[IBIS Ver]   5.0
[File name]   rzg2ul_13mm.ibs
[File Rev]   1.02
[Date]   May 27, 2025
[Source]   From silicon level SPICE model at
|   Renesas Electronics Corporation.
[Notes]
|   RZG2UL_IBIS_MODEL
|(1) This IBIS file checked the format with ibischk7.
|   Format Error are 0 and Warning are 5.
|   The 5 Warnings can be ignored.
|(2) Temperature described Tj.
|   Tj[deg]
|   Typical   25.00
|   Minimum   125.00
|   Maximum   -40.00
|(3) History
|   Rev 1.02
|   New creation by Renesas Electronics
[Disclaimer]
   These IBIS models are provided "AS IS" with no warranty and RENESAS
   is not responsible for any problems this model may cause to the customers.
   These models are subject to change without any notice.
[Copyright]   Copyright (C) 2025, Renesas Electronics Corporation. ,
|   All Rights Reserved.
[Component]   R9A07G043Ux5GBG
[Manufacturer]  Renesas Electronics Corporation.
| IBIS	DATA
| date	:	2021.9.17
| product	:	RZ/G2UL(PKG-B)
| pin   :	361pin
| printed	by	Renesas	Electronics
[Package]
|   typ   min   max
R_pkg   0.22598   0.34368   0.13006
L_pkg   3.913e-9   6.179e-9   1.918e-9
C_pkg   5.506e-13   8.624e-13   3.59e-13
[Pin]   Signal_name   model_name   R_pin   L_pin   C_pin
A9   AUDIO_CLK1   gpio_33v   0.22861   4.147e-9   4.707e-13
B8   AUDIO_CLK2   gpio_33v   0.21663   3.755e-9   5.043e-13
AE22   BSCANP   inbuf_33v   0.23766   4.548e-9   5.913e-13
AD21   VSS   inbuf_33v   0.22763   3.912e-9   4.986e-13
AE11   CSI_CLKN   AS28FMIP0000_IN   0.20128   3.731e-9   5.503e-13
AD11   CSI_CLKP   AS28FMIP0000_IN   0.18569   3.345e-9   5.496e-13
AE12   CSI_DATA0_N   AS28FMIP0000_IN   0.20766   3.838e-9   5.441e-13
AD12   CSI_DATA0_P   AS28FMIP0000_IN   0.19122   3.829e-9   5.488e-13
AE10   CSI_DATA1_N   AS28FMIP0000_IN   0.21307   4.036e-9   5.315e-13
AD10   CSI_DATA1_P   AS28FMIP0000_IN   0.19753   3.631e-9   5.495e-13
AE13   CSI_DATA2_N   AS28FMIP0000_IN   0.19175   3.578e-9   5.136e-13
AD13   CSI_DATA2_P   AS28FMIP0000_IN   0.18647   3.071e-9   4.943e-13
AE9   CSI_DATA3_N   AS28FMIP0000_IN   0.21591   3.771e-9   4.931e-13
AD9   CSI_DATA3_P   AS28FMIP0000_IN   0.19652   3.518e-9   5.449e-13
E25   DDR_ADDR0   DDR_ADRCNT   0.30852   5.269e-9   6.159e-13
K25   DDR_ADDR1   DDR_ADRCNT   0.29634   4.554e-9   5.505e-13
C25   DDR_ADDR2   DDR_ADRCNT   0.26285   5.286e-9   6.163e-13
C24   DDR_ADDR3   DDR_ADRCNT   0.28989   5.352e-9   6.454e-13
K23   DDR_ADDR4   DDR_ADRCNT   0.17693   2.994e-9   6.191e-13
B25   DDR_ADDR5   DDR_ADRCNT   0.33272   6.113e-9   6.962e-13
J25   DDR_ADDR6   DDR_ADRCNT   0.27229   4.79e-9   4.998e-13
A24   DDR_ADDR7   DDR_ADRCNT   0.34368   5.378e-9   7.14e-13
F25   DDR_ADDR8   DDR_ADRCNT   0.29546   5.204e-9   6.227e-13
B24   DDR_ADDR9   DDR_ADRCNT   0.26012   4.939e-9   7.012e-13
P23   DDR_ADDR10   DDR_ADRCNT   0.18289   2.726e-9   6.091e-13
H25   DDR_ADDR11   DDR_ADRCNT   0.22105   3.873e-9   4.949e-13
N23   DDR_ADDR12   DDR_ADRCNT   0.17797   2.693e-9   7.079e-13
D23   DDR_ADDR13   DDR_ADRCNT   0.22666   3.81e-9   5.753e-13
H23   DDR_ADDR14   DDR_ADRCNT   0.18025   2.93e-9   8.022e-13
D25   DDR_ADDR15   DDR_ADRCNT   0.29085   4.879e-9   6.257e-13
E24   DDR_BA0   DDR_ADRCNT   0.22101   3.606e-9   8.624e-13
L24   DDR_BA1   DDR_ADRCNT   0.2406   4.046e-9   5.626e-13
F23   DDR_BA2   DDR_ADRCNT   0.19749   3.016e-9   5.408e-13
A23   DDR_CALIBRATION   DDR_ADRCNT   0.27572   5.06e-9   6.049e-13
J24   DDR_CAS#   DDR_ADRCNT   0.19882   3.454e-9   5.111e-13
M25   DDR_CKE   DDR_ADRCNT   0.28365   4.337e-9   5.383e-13
P24   DDR_CLK_N   DDR_ADRCNT   0.2062   3.263e-9   4.953e-13
P25   DDR_CLK_P   DDR_ADRCNT   0.22344   3.65e-9   5.223e-13
N24   DDR_CS0#   DDR_ADRCNT   0.26763   3.955e-9   4.808e-13
L23   DDR_CS1#   DDR_ADRCNT   0.17047   2.819e-9   5.72e-13
U23   DDR_DM0   DDR_DQDMDQS   0.18554   2.794e-9   6.509e-13
Y24   DDR_DM1   DDR_DQDMDQS   0.28328   4.288e-9   6.595e-13
T25   DDR_DQ0   DDR_DQDMDQS   0.2478   4.283e-9   5.606e-13
W24   DDR_DQ1   DDR_DQDMDQS   0.23177   3.721e-9   4.888e-13
R24   DDR_DQ2   DDR_DQDMDQS   0.21916   3.48e-9   4.656e-13
Y25   DDR_DQ3   DDR_DQDMDQS   0.32654   4.752e-9   5.881e-13
T24   DDR_DQ4   DDR_DQDMDQS   0.27525   3.952e-9   5.711e-13
U25   DDR_DQ5   DDR_DQDMDQS   0.26125   4.103e-9   4.181e-13
R25   DDR_DQ6   DDR_DQDMDQS   0.28132   4.458e-9   4.363e-13
T23   DDR_DQ7   DDR_DQDMDQS   0.18032   2.637e-9   4.866e-13
AD24   DDR_DQ8   DDR_DQDMDQS   0.32838   4.655e-9   6.905e-13
AA24   DDR_DQ9   DDR_DQDMDQS   0.2742   4.67e-9   5.683e-13
W23   DDR_DQ10   DDR_DQDMDQS   0.18485   2.966e-9   4.618e-13
AD25   DDR_DQ11   DDR_DQDMDQS   0.27727   4.493e-9   7.8e-13
AD23   DDR_DQ12   DDR_DQDMDQS   0.25366   4.031e-9   7.58e-13
AA23   DDR_DQ13   DDR_DQDMDQS   0.20546   3.203e-9   7.392e-13
AC24   DDR_DQ14   DDR_DQDMDQS   0.30091   4.578e-9   7.764e-13
AE24   DDR_DQ15   DDR_DQDMDQS   0.33205   4.835e-9   5.793e-13
V24   DDR_DQS0_N   DDR_DQDMDQS   0.2145   3.127e-9   7.214e-13
V25   DDR_DQS0_P   DDR_DQDMDQS   0.23258   3.363e-9   6.777e-13
AB25   DDR_DQS1_N   DDR_DQDMDQS   0.26811   4.843e-9   6.631e-13
AB24   DDR_DQS1_P   DDR_DQDMDQS   0.27051   4.409e-9   7.234e-13
M24   DDR_ODT0   DDR_ADRCNT   0.22209   3.696e-9   5.376e-13
L25   DDR_ODT1   DDR_ADRCNT   0.27722   4.972e-9   5.408e-13
H24   DDR_RAS#   DDR_ADRCNT   0.26066   4.61e-9   5.523e-13
B23   DDR_RESET#   DDR_ADRCNT   0.31098   5.139e-9   6.32e-13
G25   DDR_WE#   DDR_ADRCNT   0.24637   4.632e-9   5.755e-13
Y19   DEBUGEN   inbuf_33v   0.15054   2.54e-9   6.669e-13
A10   DISP_CLK   gpio_33v   0.19853   3.939e-9   4.928e-13
B10   DISP_DATA0   gpio_33v   0.20629   3.552e-9   4.659e-13
A11   DISP_DATA1   gpio_33v   0.23075   3.819e-9   4.912e-13
B11   DISP_DATA2   gpio_33v   0.21122   3.381e-9   4.594e-13
A12   DISP_DATA3   gpio_33v   0.23395   3.581e-9   4.354e-13
B12   DISP_DATA4   gpio_33v   0.17421   3.057e-9   4.43e-13
C11   DISP_DATA5   gpio_33v   0.15695   2.26e-9   4.267e-13
C12   DISP_DATA6   gpio_33v   0.19989   3.05e-9   5.531e-13
C13   DISP_DATA7   gpio_33v   0.19809   3.019e-9   4.691e-13
A13   DISP_DATA8   gpio_33v   0.22642   3.908e-9   4.72e-13
B13   DISP_DATA9   gpio_33v   0.18059   3.095e-9   4.947e-13
A14   DISP_DATA10   gpio_33v   0.22656   3.822e-9   4.855e-13
C14   DISP_DATA11   gpio_33v   0.14189   2.292e-9   5.438e-13
B14   DISP_DATA12   gpio_33v   0.20803   3.339e-9   4.987e-13
C15   DISP_DATA13   gpio_33v   0.19625   3.149e-9   5.702e-13
A15   DISP_DATA14   gpio_33v   0.22045   3.914e-9   5.069e-13
F16   DISP_DATA15   gpio_33v   0.13006   1.918e-9   4.682e-13
B15   DISP_DATA16   gpio_33v   0.17178   3.267e-9   4.714e-13
C16   DISP_DATA17   gpio_33v   0.13851   2.371e-9   4.245e-13
A16   DISP_DATA18   gpio_33v   0.22064   3.986e-9   5.073e-13
B16   DISP_DATA19   gpio_33v   0.19052   3.137e-9   4.751e-13
A17   DISP_DATA20   gpio_33v   0.22782   4.166e-9   5.222e-13
B17   DISP_DATA21   gpio_33v   0.20624   3.572e-9   4.594e-13
C17   DISP_DATA22   gpio_33v   0.20862   3.611e-9   5.4e-13
C20   DISP_DATA23   gpio_33v   0.21051   3.694e-9   4.442e-13
C9   DISP_DE   gpio_33v   0.15116   2.627e-9   4.184e-13
B9   DISP_HSYNC   gpio_33v   0.2102   3.714e-9   4.29e-13
C10   DISP_VSYNC   gpio_33v   0.20786   3.501e-9   4.613e-13
P1   ET0_LINKSTA   rgmii_RIP_BI_SDS_1833V_NC   0.23928   4.222e-9   5.233e-13
T3   ET0_MDC   rgmii_RIP_BI_SDS_1833V_NC   0.21992   3.494e-9   5.227e-13
T2   ET0_MDIO   rgmii_RIP_BI_SDS_1833V_NC   0.21286   3.468e-9   5.939e-13
N3   ET0_RXC/RX_CLK   rgmii_RIP_BI_SDS_1833V_NC   0.21486   3.382e-9   5.835e-13
P2   ET0_RXD0   rgmii_RIP_BI_SDS_1833V_NC   0.1839   3.418e-9   4.518e-13
R3   ET0_RXD1   rgmii_RIP_BI_SDS_1833V_NC   0.21332   3.578e-9   5.481e-13
R2   ET0_RXD2   rgmii_RIP_BI_SDS_1833V_NC   0.22457   3.76e-9   5.597e-13
R1   ET0_RXD3   rgmii_RIP_BI_SDS_1833V_NC   0.23988   4.317e-9   5.185e-13
N1   ET0_RX_CTL/RX_DV   rgmii_RIP_BI_SDS_1833V_NC   0.23729   4.049e-9   5.049e-13
N2   ET0_RX_ERR   rgmii_RIP_BI_SDS_1833V_NC   0.21881   3.664e-9   4.935e-13
M2   ET0_TXC/TX_CLK   rgmii_RIP_BI_SDS_1833V_NC   0.20357   3.313e-9   4.826e-13
L1   ET0_TXD0   rgmii_RIP_BI_SDS_1833V_NC   0.24019   4.155e-9   5.204e-13
L2   ET0_TXD1   rgmii_RIP_BI_SDS_1833V_NC   0.22097   3.526e-9   5.78e-13
K1   ET0_TXD2   rgmii_RIP_BI_SDS_1833V_NC   0.23897   4.163e-9   5.179e-13
K2   ET0_TXD3   rgmii_RIP_BI_SDS_1833V_NC   0.22361   3.659e-9   5.463e-13
M3   ET0_TX_COL   rgmii_RIP_BI_SDS_1833V_NC   0.13984   2.506e-9   4.252e-13
M6   ET0_TX_CRS   rgmii_RIP_BI_SDS_1833V_NC   0.13124   2.049e-9   4.926e-13
M1   ET0_TX_CTL/TX_EN   rgmii_RIP_BI_SDS_1833V_NC   0.23547   4.139e-9   5.272e-13
K6   ET0_TX_ERR   rgmii_RIP_BI_SDS_1833V_NC   0.2133   3.521e-9   5.968e-13
AC19   ET1_LINKSTA   rgmii_RIP_BI_SDS_1833V_NC   0.21229   3.367e-9   5.938e-13
AC20   ET1_MDC   rgmii_RIP_BI_SDS_1833V_NC   0.19485   3.192e-9   4.294e-13
AE21   ET1_MDIO   rgmii_RIP_BI_SDS_1833V_NC   0.24993   4.505e-9   5.2e-13
AC17   ET1_RXC/RX_CLK   rgmii_RIP_BI_SDS_1833V_NC   0.19068   3.173e-9   5.904e-13
AE19   ET1_RXD0   rgmii_RIP_BI_SDS_1833V_NC   0.2318   4.258e-9   5.507e-13
AD19   ET1_RXD1   rgmii_RIP_BI_SDS_1833V_NC   0.21543   3.788e-9   5.39e-13
AE20   ET1_RXD2   rgmii_RIP_BI_SDS_1833V_NC   0.23799   4.307e-9   5.456e-13
AD20   ET1_RXD3   rgmii_RIP_BI_SDS_1833V_NC   0.22453   3.747e-9   5.686e-13
AC18   ET1_RX_CTL/RX_DV   rgmii_RIP_BI_SDS_1833V_NC   0.14167   2.338e-9   4.536e-13
AD18   ET1_RX_ERR   rgmii_RIP_BI_SDS_1833V_NC   0.2107   3.683e-9   5.402e-13
AE18   ET1_TXC/TX_CLK   rgmii_RIP_BI_SDS_1833V_NC   0.22618   4.132e-9   4.835e-13
AD16   ET1_TXD0   rgmii_RIP_BI_SDS_1833V_NC   0.1911   3.153e-9   4.595e-13
AE16   ET1_TXD1   rgmii_RIP_BI_SDS_1833V_NC   0.22095   4.002e-9   4.821e-13
AD15   ET1_TXD2   rgmii_RIP_BI_SDS_1833V_NC   0.20437   3.453e-9   4.809e-13
AE15   ET1_TXD3   rgmii_RIP_BI_SDS_1833V_NC   0.20919   3.458e-9   4.123e-13
AC16   ET1_TX_COL   rgmii_RIP_BI_SDS_1833V_NC   0.1327   2.314e-9   4.305e-13
AC15   ET1_TX_CRS   rgmii_RIP_BI_SDS_1833V_NC   0.14353   2.264e-9   4.933e-13
AD17   ET1_TX_CTL/TX_EN   rgmii_RIP_BI_SDS_1833V_NC   0.20566   3.594e-9   4.827e-13
AE17   ET1_TX_ERR   rgmii_RIP_BI_SDS_1833V_NC   0.22147   4.045e-9   4.995e-13
Y3   EXCLK   inbuf_33v   0.18247   2.935e-9   4.861e-13
B22   IRQ6   gpio_33v   0.238   4.391e-9   4.568e-13
A21   IRQ7   gpio_33v   0.22295   4.52e-9   5.478e-13
G6   MD_BOOT0   inbuf_33v   0.17061   2.786e-9   5.253e-13
C5   MD_BOOT1   inbuf_33v   0.20696   3.408e-9   4.625e-13
C4   MD_BOOT2   inbuf_33v   0.21541   3.666e-9   4.748e-13
F20   MD_CLKS   inbuf_33v   0.20617   3.517e-9   5.444e-13
A22   MD_OSCDRV0   inbuf_33v   0.25713   4.841e-9   5.306e-13
C21   MD_OSCDRV1   inbuf_33v   0.17909   3.207e-9   3.792e-13
AA2   NMI   gpio_33v   0.23155   4.205e-9   7.23e-13
B2   NC   sdio_STP_BI_016_1833V_SD3   0.26124   4.797e-9   5.818e-13
A4   NC   sdio_STP_BI_016_1833V_SD3   0.26691   5.034e-9   5.827e-13
B4   NC   sdio_STP_BI_016_1833V_SD3   0.25349   4.576e-9   6.25e-13
A3   NC   sdio_STP_BI_016_1833V_SD3   0.25227   4.987e-9   5.937e-13
B3   NC   sdio_STP_BI_016_1833V_SD3   0.26984   4.809e-9   6.384e-13
A2   NC   sdio_STP_BI_016_1833V_SD3   0.29359   5.578e-9   6.773e-13
AC3   P5_1   gpio_33v   0.16462   3.407e-9   4.695e-13
AB2   P6_2   gpio_33v   0.27733   6.179e-9   5.998e-13
AC1   P6_3   gpio_33v   0.25661   5.108e-9   5.885e-13
AC2   P6_4   gpio_33v   0.23412   3.923e-9   6.024e-13
W2   PRST#   gpio_33v   0.13355   3.131e-9   5.388e-13
C7   QSPI0_IO0   sdio_STP_BI_016_1833V_SD3   0.21696   3.457e-9   5.407e-13
A5   QSPI0_IO1   sdio_STP_BI_016_1833V_SD3   0.25155   4.652e-9   5.678e-13
B7   QSPI0_IO2   sdio_STP_BI_016_1833V_SD3   0.22587   3.789e-9   5.737e-13
C6   QSPI0_IO3   sdio_STP_BI_016_1833V_SD3   0.22339   3.646e-9   5.416e-13
B6   QSPI0_SPCLK   sdio_STP_BI_016_1833V_SD3   0.20303   3.787e-9   5.345e-13
B5   QSPI0_SSL   sdio_STP_BI_016_1833V_SD3   0.24229   4.387e-9   5.664e-13
A7   QSPI_RESET#   sdio_STP_BI_016_1833V_SD3   0.24456   4.339e-9   5.523e-13
A6   QSPI_WP#   sdio_STP_BI_016_1833V_SD3   0.25587   4.507e-9   5.749e-13
B19   RIIC0_SCL   iic_33v   0.20428   3.35e-9   4.125e-13
B20   RIIC0_SDA   iic_33v   0.23614   3.967e-9   5.251e-13
A19   RIIC1_SCL   iic_33v   0.24373   4.293e-9   4.502e-13
A20   RIIC1_SDA   iic_33v   0.25488   4.429e-9   5.437e-13
B1   SD0_CD   gpio_33v   0.27618   5.469e-9   6.12e-13
G1   SD0_CLK   sdio_STP_BI_016_1833V_SD3   0.26669   4.94e-9   5.992e-13
E2   SD0_CMD   sdio_STP_BI_016_1833V_SD3   0.24036   4.423e-9   5.822e-13
F1   SD0_DATA0   sdio_STP_BI_016_1833V_SD3   0.28096   5.207e-9   5.788e-13
H3   SD0_DATA1   sdio_STP_BI_016_1833V_SD3   0.21572   3.747e-9   7.649e-13
F2   SD0_DATA2   sdio_STP_BI_016_1833V_SD3   0.23704   4.353e-9   6.061e-13
D2   SD0_DATA3   sdio_STP_BI_016_1833V_SD3   0.22699   4.002e-9   6.391e-13
E1   SD0_DATA4   sdio_STP_BI_016_1833V_SD3   0.252   4.728e-9   6.238e-13
D1   SD0_DATA5   sdio_STP_BI_016_1833V_SD3   0.25925   4.933e-9   5.889e-13
E3   SD0_DATA6   sdio_STP_BI_016_1833V_SD3   0.22365   3.793e-9   7.306e-13
F3   SD0_DATA7   sdio_STP_BI_016_1833V_SD3   0.2175   3.618e-9   5.977e-13
C1   SD0_RST#   sdio_STP_BI_016_1833V_SD3   0.2641   5.004e-9   6.63e-13
C2   SD0_WP   gpio_33v   0.25951   4.981e-9   5.668e-13
D3   SD1_CD   gpio_33v   0.21151   3.733e-9   5.544e-13
G2   SD1_CLK   sdio_STP_BI_016_1833V_SD3   0.2266   3.877e-9   5.907e-13
H6   SD1_CMD   sdio_STP_BI_016_1833V_SD3   0.21716   3.71e-9   7.013e-13
H2   SD1_DATA0   sdio_STP_BI_016_1833V_SD3   0.23134   3.903e-9   5.261e-13
J3   SD1_DATA1   sdio_STP_BI_016_1833V_SD3   0.15703   2.653e-9   5.032e-13
J1   SD1_DATA2   sdio_STP_BI_016_1833V_SD3   0.23838   4.194e-9   5.026e-13
J2   SD1_DATA3   sdio_STP_BI_016_1833V_SD3   0.22062   3.657e-9   5.246e-13
C3   SD1_WP   gpio_33v   0.18174   3.832e-9   5.818e-13
U2   TCK/SWDCLK   inbuf_18v   0.23262   3.792e-9   3.996e-13
W1   TDI   inbuf_18v   0.26173   4.632e-9   5.884e-13
V2   TDO   gpio_18v   0.23571   3.957e-9   5.511e-13
AD22   VSS   inbuf_33v   0.24153   4.382e-9   4.981e-13
U1   TMS/SWDIO   gpio_18v   0.24779   4.278e-9   5.03e-13
V1   TRST#   inbuf_18v   0.22355   4.318e-9   5.309e-13
AE6   USB0_DM   as28fus20002vwbp1hs_dm   0.23395   3.919e-9   5.907e-13
AD6   USB0_DP   as28fus20002vwbp1hs_dp   0.21645   3.683e-9   6.102e-13
AB3   USB0_OTG_EXICEN   gpio_33v   0.21864   3.991e-9   6.97e-13
AD2   USB0_OTG_ID   gpio_33v   0.25189   4.972e-9   6.132e-13
AE3   USB0_OVRCUR   gpio_33v   0.26986   5.24e-9   6.012e-13
AD3   USB0_VBUSEN   gpio_33v   0.24994   4.648e-9   5.443e-13
AD8   USB0_VBUSIN   iic_33v   0.2033   3.727e-9   3.59e-13
AE5   USB1_DM   as28fus20002vwbp1hs_dm   0.24031   3.992e-9   5.792e-13
AD5   USB1_DP   as28fus20002vwbp1hs_dp   0.23092   3.546e-9   6.05e-13
AE2   USB1_OVRCUR   gpio_33v   0.23373   5.484e-9   6.009e-13
AD1   USB1_VBUSEN   gpio_33v   0.29109   5.779e-9   7.063e-13
B21   WDTOVF_PERROUT#   gpio_33v   0.20442   3.983e-9   5.655e-13
[Series Pin Mapping]   pin_2   model_name
AD11 AE11 AS28FMIP0000_TERM
AD12 AE12 AS28FMIP0000_TERM
AD10 AE10 AS28FMIP0000_TERM
AD13 AE13 AS28FMIP0000_TERM
AD9 AE9 AS28FMIP0000_TERM
[Diff Pin] inv_pin   vdiff   tdelay_typ   tdelay_min   tdelay_max
| The '+' pin is Diff_pin and the '-' pin is the inv_pin
| Receiver Vth = +/-100mV
|PAD_P   PAD_N   0.07   0   0   0
AD11 AE11 0.07 0 0 0
AD12 AE12 0.07 0 0 0
AD10 AE10 0.07 0 0 0
AD13 AE13 0.07 0 0 0
AD9 AE9 0.07 0 0 0
|[Diff pin]  inv_pin  vdiff   tdelay_typ   tdelay_min   tdelay_max
|DP   DM   100.000mV  0.0s   0.0s   0.0s
AD6 AE6 100mV 0 0 0
AD5 AE5 100mV 0 0 0
[Model Selector] gpio_33v
gpio_33v_12m_fast  SRP_BI_SDS_33V_STB_33V_e2e1_11_SR1
gpio_33v_12m_slow  SRP_BI_SDS_33V_STB_33V_e2e1_11_SR0
gpio_33v_2m_fast   SRP_BI_SDS_33V_STB_33V_e2e1_00_SR1
gpio_33v_2m_slow   SRP_BI_SDS_33V_STB_33V_e2e1_00_SR0
gpio_33v_4m_fast   SRP_BI_SDS_33V_STB_33V_e2e1_01_SR1
gpio_33v_4m_slow   SRP_BI_SDS_33V_STB_33V_e2e1_01_SR0
gpio_33v_8m_fast   SRP_BI_SDS_33V_STB_33V_e2e1_10_SR1
gpio_33v_8m_slow   SRP_BI_SDS_33V_STB_33V_e2e1_10_SR0
[Model Selector] gpio_18v
gpio_18v_12m_fast  SRP_BI_SDS_33V_STB_18V_e2e1_11_SR1
gpio_18v_12m_slow  SRP_BI_SDS_33V_STB_18V_e2e1_11_SR0
gpio_18v_2m_fast   SRP_BI_SDS_33V_STB_18V_e2e1_00_SR1
gpio_18v_2m_slow   SRP_BI_SDS_33V_STB_18V_e2e1_00_SR0
gpio_18v_4m_fast   SRP_BI_SDS_33V_STB_18V_e2e1_01_SR1
gpio_18v_4m_slow   SRP_BI_SDS_33V_STB_18V_e2e1_01_SR0
gpio_18v_8m_fast   SRP_BI_SDS_33V_STB_18V_e2e1_10_SR1
gpio_18v_8m_slow   SRP_BI_SDS_33V_STB_18V_e2e1_10_SR0
[Model Selector] sdio_STP_BI_016_1833V_SD3
sdio_18v_33_fast   STP_BI_016_1833V_SD3_18V_e2e1_00_SR0
sdio_18v_33_slow   STP_BI_016_1833V_SD3_18V_e2e1_00_SR0
sdio_18v_50_fast   STP_BI_016_1833V_SD3_18V_e2e1_01_SR0
sdio_18v_50_slow   STP_BI_016_1833V_SD3_18V_e2e1_01_SR0
sdio_18v_66_fast   STP_BI_016_1833V_SD3_18V_e2e1_10_SR0
sdio_18v_66_slow   STP_BI_016_1833V_SD3_18V_e2e1_10_SR0
sdio_18v_100_fast  STP_BI_016_1833V_SD3_18V_e2e1_11_SR0
sdio_18v_100_slow  STP_BI_016_1833V_SD3_18V_e2e1_11_SR0
sdio_33v_5_fast   STP_BI_016_1833V_SD3_33V_e2e1_11_SR0
sdio_33v_5_slow   STP_BI_016_1833V_SD3_33V_e2e1_11_SR0
sdio_33v_12_fast  STP_BI_016_1833V_SD3_33V_e2e1_10_SR0
sdio_33v_12_slow  STP_BI_016_1833V_SD3_33V_e2e1_10_SR0
sdio_33v_26_fast  STP_BI_016_1833V_SD3_33V_e2e1_01_SR0
sdio_33v_26_slow  STP_BI_016_1833V_SD3_33V_e2e1_01_SR0
sdio_33v_40_fast  STP_BI_016_1833V_SD3_33V_e2e1_00_SR0
sdio_33v_40_slow  STP_BI_016_1833V_SD3_33V_e2e1_00_SR0
[Model Selector] rgmii_RIP_BI_SDS_1833V_NC
rgmii_18v   RIP_BI_SDS_1833V_NC_18
rgmii_25v   RIP_BI_SDS_1833V_NC_25
rgmii_33v   RIP_BI_SDS_1833V_NC_33
[Model Selector] DDR_ADRCNT
PAD_60_0_USEIO_ddr4_0p5   Z0=60-Ohm Driver   ODT disable
PAD_60_0_USEIO_ddr3l   Z0=60-Ohm Driver   ODT disable
PAD_60_0_USEIO_ddr3   Z0=60-Ohm Driver   ODT disable
[Model Selector] DDR_DQDMDQS
PAD_40_120_USEIO_ddr4_0p8   Z0=40-Ohm Driver   120-Ohm Pull-up
PAD_40_80_USEIO_ddr4_0p8   Z0=40-Ohm Driver   80-Ohm Pull-up
PAD_40_60_USEIO_ddr4_0p8   Z0=40-Ohm Driver   60-Ohm Pull-up
PAD_40_48_USEIO_ddr4_0p8   Z0=40-Ohm Driver   48-Ohm Pull-up
PAD_40_40_USEIO_ddr4_0p8   Z0=40-Ohm Driver   40-Ohm Pull-up
PAD_34_0_USEIO_ddr4_0p8   Z0=34-Ohm Driver   ODT disable
PAD_48_0_USEIO_ddr4_0p8   Z0=48-Ohm Driver   ODT disable
PAD_60_0_USEIO_ddr4_0p8   Z0=60-Ohm Driver   ODT disable
PAD_40_120_USEIO_ddr3l   Z0=40-Ohm Driver   120-Ohm equivalent termination
PAD_40_60_USEIO_ddr3l   Z0=40-Ohm Driver   60-Ohm equivalent termination
PAD_40_40_USEIO_ddr3l   Z0=40-Ohm Driver   40-Ohm equivalent termination
PAD_34_0_USEIO_ddr3l   Z0=34-Ohm Driver   ODT disable
PAD_48_0_USEIO_ddr3l   Z0=48-Ohm Driver   ODT disable
PAD_60_0_USEIO_ddr3l   Z0=60-Ohm Driver   ODT disable
PAD_40_120_USEIO_ddr3   Z0=40-Ohm Driver   120-Ohm equivalent termination
PAD_40_60_USEIO_ddr3   Z0=40-Ohm Driver   60-Ohm equivalent termination
PAD_40_40_USEIO_ddr3   Z0=40-Ohm Driver   40-Ohm equivalent termination
PAD_34_0_USEIO_ddr3   Z0=34-Ohm Driver   ODT disable
PAD_48_0_USEIO_ddr3   Z0=48-Ohm Driver   ODT disable
PAD_60_0_USEIO_ddr3   Z0=60-Ohm Driver   ODT disable
|   Model AS28FMIP0000_TERM
[Model]   AS28FMIP0000_TERM
Model_type   Series
Polarity   Non-Inverting
C_comp   0.0pF   0.0pF   0.0pF
[Temperature Range] 25   125   -40
[Voltage Range]   1.8   1.65   1.95
| Resistance   ohm(typ)   ohm(min)   ohm(max)
[R Series]   100   80   125
| Models and submodels in the file (342): gpio_33v_12m_fast (I/O), gpio_33v_12m_slow (I/O), gpio_33v_2m_fast (I/O), gpio_33v_2m_slow (I/O), gpio_33v_4m_fast (I/O), gpio_33v_4m_slow (I/O), gpio_33v_8m_fast (I/O), gpio_33v_8m_slow (I/O), gpio_18v_12m_fast (I/O), gpio_18v_12m_slow (I/O), gpio_18v_2m_fast (I/O), gpio_18v_2m_slow (I/O), gpio_18v_4m_fast (I/O), gpio_18v_4m_slow (I/O), gpio_18v_8m_fast (I/O), gpio_18v_8m_slow (I/O), sdio_18v_33_fast (I/O), sdio_18v_33_slow (I/O), sdio_18v_50_fast (I/O), sdio_18v_50_slow (I/O), sdio_18v_66_fast (I/O), sdio_18v_66_slow (I/O), sdio_18v_100_fast (I/O), sdio_18v_100_slow (I/O), sdio_33v_5_fast (I/O), sdio_33v_5_slow (I/O), sdio_33v_12_fast (I/O), sdio_33v_12_slow (I/O), sdio_33v_26_fast (I/O), sdio_33v_26_slow (I/O), sdio_33v_40_fast (I/O), sdio_33v_40_slow (I/O), rgmii_18v (I/O), rgmii_25v (I/O), rgmii_33v (I/O), iic_33v (I/O_open_drain), inbuf_18v (Input), inbuf_33v (Input), AS28FMIP0000_IN (Input), as28fus20002vwbp1hs_dp (I/O), as28fus20002vwbp1hs_dm (I/O), AS28FMIP0000_TERM (Series), PAD_60_0_USEIO_ddr3 (I/O), PAD_60_120_USEIO_ddr3 (I/O), PAD_60_120_ddr3_T (Dynamic_clamp), PAD_60_60_USEIO_ddr3 (I/O), PAD_60_60_ddr3_T (Dynamic_clamp), PAD_60_40_USEIO_ddr3 (I/O), PAD_60_40_ddr3_T (Dynamic_clamp), PAD_60_30_USEIO_ddr3 (I/O), PAD_60_30_ddr3_T (Dynamic_clamp), PAD_60_24_USEIO_ddr3 (I/O), PAD_60_24_ddr3_T (Dynamic_clamp), PAD_60_20_USEIO_ddr3 (I/O), PAD_60_20_ddr3_T (Dynamic_clamp), PAD_60_17_USEIO_ddr3 (I/O), PAD_60_17_ddr3_T (Dynamic_clamp), PAD_48_0_USEIO_ddr3 (I/O), PAD_48_120_USEIO_ddr3 (I/O), PAD_48_120_ddr3_T (Dynamic_clamp), PAD_48_60_USEIO_ddr3 (I/O), PAD_48_60_ddr3_T (Dynamic_clamp), PAD_48_40_USEIO_ddr3 (I/O), PAD_48_40_ddr3_T (Dynamic_clamp), PAD_48_30_USEIO_ddr3 (I/O), PAD_48_30_ddr3_T (Dynamic_clamp), PAD_48_24_USEIO_ddr3 (I/O), PAD_48_24_ddr3_T (Dynamic_clamp), PAD_48_20_USEIO_ddr3 (I/O), PAD_48_20_ddr3_T (Dynamic_clamp), PAD_48_17_USEIO_ddr3 (I/O), PAD_48_17_ddr3_T (Dynamic_clamp), PAD_40_0_USEIO_ddr3 (I/O), PAD_40_120_USEIO_ddr3 (I/O), PAD_40_120_ddr3_T (Dynamic_clamp), PAD_40_60_USEIO_ddr3 (I/O), PAD_40_60_ddr3_T (Dynamic_clamp), PAD_40_40_USEIO_ddr3 (I/O), PAD_40_40_ddr3_T (Dynamic_clamp), PAD_40_30_USEIO_ddr3 (I/O)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
